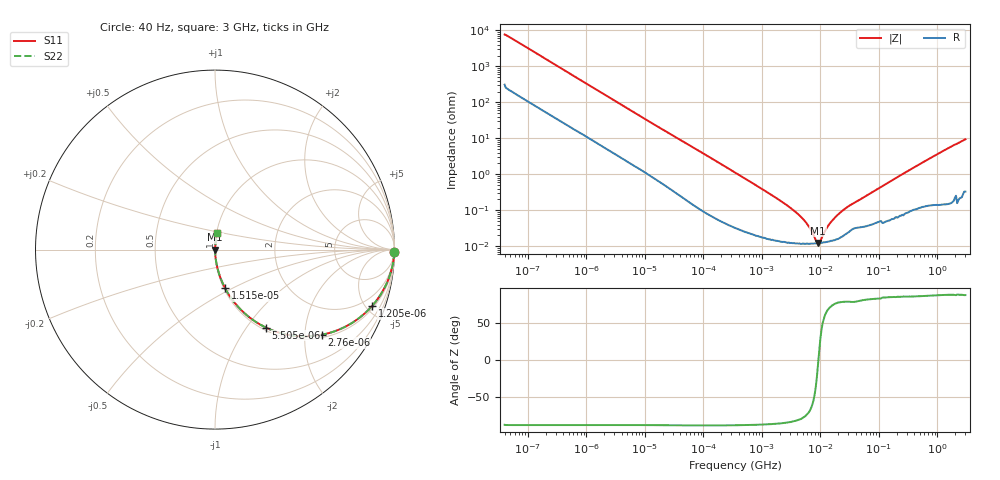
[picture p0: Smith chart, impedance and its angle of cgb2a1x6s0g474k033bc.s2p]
! S-parameter Generated by TDK Corporation
! Copyright(C) 2015 TDK Corporation.
! All Rights Reserved.
! TDK P/N: CGB2A1X6S0G474K033BC (Multilayer Ceramic Chip Capacitors)
! Property: C=470nF
! Size(LxWxT): 1x0.5x0.33mm, 0.039x0.02x0.013inches
! Model Type: s2p (Touchstone File Format Version 1.0)
! Frequency: DC=Yes Start=0.00004MHz Stop=3000MHz 396points Log-sweep
! Note: This model was converted from impedance.
! Model Generated on Jun. 23, 2015
! Hash(MD5):
! Port Assignments:
!  1 ---| |--- 2
! Applicable Conditions:
!  Temperature = 25 degC
!  DC Bias Voltage = 0 V
!  Small Signal Operation
! Terms and conditions regarding TDK Simulation Models
! (1)This simulation model is being provided solely for informational purposes. Please refer to the specifications of the products in terms of detailed characteristics of such products.
! (2)In no event shall TDK Corporation of any of its subsidiaries be liable for any loss or damage arising, directly or indirectly,
!  From any information contained in this simulation model, including, but not limited to loss or damages arising from any inaccuracies, omissions or errors in connection with such information.
! (3)Any and all copyrights on this simulation model are owned by TDK Corporation.
!  Duplication or redistribution of this simulation model without prior written permission from TDK Corporation is prohibited.
! (4)This simulation model is subject to any modification or change without any prior notice.
! (5)Neither TDK Corporation nor any of its subsidiaries shall make any warranty, express or implied,
!  Including but not limited to the correctness, implied warranties of merchantability and fitness for a particular purpose with respect to this simulation models.
! (6)The use of this simulation model shall be deemed to have consented to the terms and conditions hereof.
# MHz S MA R 50
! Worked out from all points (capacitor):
!   395 points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, 40 Hz to 3 GHz, reference 50 ohm
!   read as one part in series: C = 503 nF near 41.88 Hz
!   lowest |Z| = 12.3 mohm at 9.093 MHz (marker M1)
!   series resonance near 9.206 MHz, so ESL is about 590 pH
!   S11 on the Smith chart (normalised r, x): 40 Hz: open; 1.205 kHz: 1.18, -5.51; 2.76 kHz: 1.08, -2.43; 5.505 kHz: 1.04, -1.24; 15.15 kHz: 1.01, -0.46; 3 GHz: 1.01, +0.19
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4e-05  0.9994 -0.7  0.01296 87.0  0.01296 87.0  0.9994 -0.7
0.0002407527  0.9949 -4.2  0.07355 83.9  0.07355 83.9  0.9949 -4.2
0.000834128  0.9621 -14.0  0.2426 74.1  0.2426 74.1  0.9621 -14.0
0.001205403  0.9302 -19.7  0.3374 68.4  0.3374 68.4  0.9302 -19.7
0.002759985  0.7605 -38.6  0.6244 49.5  0.6244 49.5  0.7605 -38.6
0.005504511  0.5182 -56.9  0.8383 31.2  0.8383 31.2  0.5182 -56.9
0.008721545  0.3628 -66.9  0.92 21.3  0.92 21.3  0.3628 -66.9
0.01515106  0.2234 -75.3  0.9677 12.9  0.9677 12.9  0.2234 -75.3
0.01739424  0.1969 -76.9  0.9743 11.4  0.9743 11.4  0.1969 -76.9
0.05755453  0.06411 -84.9  0.9963 3.7  0.9963 3.7  0.06411 -84.9
0.3464102  0.01124 -87.7  0.9996 0.6  0.9996 0.6  0.01124 -87.7
3.303516  0.001068 -83.4  0.9999 0.1  0.9999 0.1  0.001068 -83.4
5.234209  0.0005336 -77.2  0.9999 0.0  0.9999 0.0  0.0005336 -77.2
7.22376  0.0002457 -60.9  0.9999 0.0  0.9999 0.0  0.0002457 -60.9
8.293268  0.0001506 -37.4  0.9999 0.0  0.9999 0.0  0.0001506 -37.4
9.092863  0.0001231 -5.3  0.9999 0.0  0.9999 0.0  0.0001231 -5.3
9.969551  0.0001419 29.1  0.9999 -0.0  0.9999 -0.0  0.0001419 29.1
13.75903  0.0003857 69.3  0.9999 -0.0  0.9999 -0.0  0.0003857 69.3
21.8003  0.0008654 78.4  0.9998 -0.0  0.9998 -0.0  0.0008654 78.4
31.50375  0.001359 78.9  0.9997 -0.1  0.9997 -0.1  0.001359 78.9
150.6385  0.006168 84.8  0.9995 -0.4  0.9995 -0.4  0.006168 84.8
3000  0.09342 82.6  0.9924 -5.4  0.9924 -5.4  0.09342 82.6
